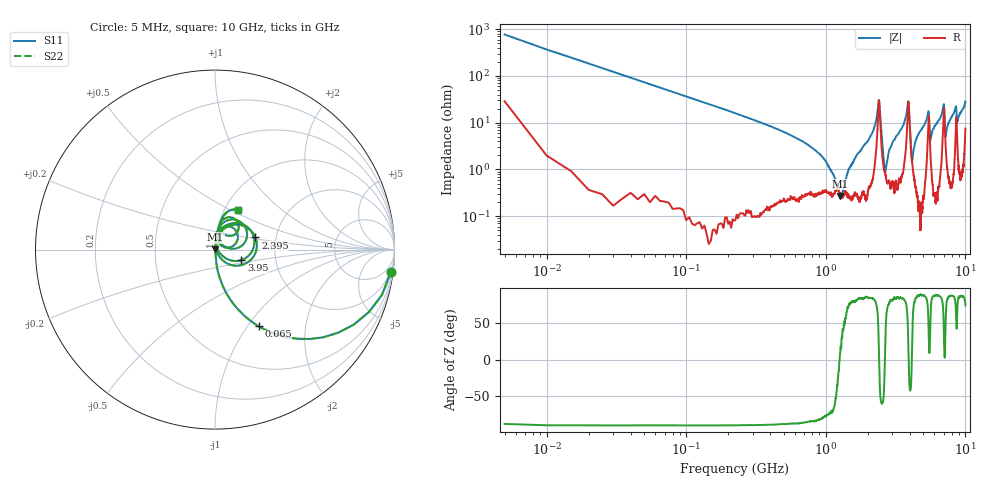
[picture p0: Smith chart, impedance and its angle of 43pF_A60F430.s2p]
! Amotech Co.,Ltd.
! http://www.amotech.co.kr/
! Part Number: A60F430
! These Parameters are Measured in Series Mode Connection
! Operation Temp=25[degC], DC Bias Voltage=0[V]
! Freq. Start=5[MHz] Stop=10[GHz], 2000[Steps]
! Date: Monday, July 20, 2020, 03:41:23
# GHZ S RI R 50.000000
!Freq.(Hz) S11(Real) S11(Imag) S21(Real) S21(Imag) S12(Real) S12(Imag) S22(Real) S22(Imag)
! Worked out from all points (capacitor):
!   2000 points, 5 MHz to 10 GHz, reference 50 ohm
!   read as one part in series: C = 43.3 pF near 55 MHz
!   lowest |Z| = 271 mohm at 1.27 GHz (marker M1)
!   series resonance near 1.256 GHz, so ESL is about 370 pH
!   S11 on the Smith chart (normalised r, x): 5 MHz: 2, -15; 65 MHz: 1.00, -1.13; 2.395 GHz: 1.56, +0.22; 3.95 GHz: 1.33, -0.16; 10 GHz: 1.15, +0.55
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0.005  0.9789 -0.1264  0.0211 0.1264  0.0211 0.1264  0.9789 -0.1264
0.065  0.2424 -0.4267  0.7576 0.4267  0.7576 0.4267  0.2424 -0.4267
0.22  0.0267 -0.1586  0.9733 0.1586  0.9733 0.1586  0.0267 -0.1586
0.955  0.00364 -0.0176  0.9964 0.0176  0.9964 0.0176  0.00364 -0.0176
1.27  0.00264 0.000585  0.9974 -0.000585  0.9974 -0.000585  0.00264 0.000585
1.675  0.00329 0.0204  0.9967 -0.0204  0.9967 -0.0204  0.00329 0.0204
2.395  0.2256 0.0676  0.7744 -0.0676  0.7744 -0.0676  0.2256 0.0676
2.66  0.00823 0.00204  0.9918 -0.00204  0.9918 -0.00204  0.00823 0.00204
2.875  0.00562 0.0271  0.9944 -0.0271  0.9944 -0.0271  0.00562 0.0271
3.34  0.01 0.0595  0.99 -0.0595  0.99 -0.0595  0.01 0.0595
3.87  0.1755 0.1293  0.8245 -0.1293  0.8245 -0.1293  0.1755 0.1293
3.95  0.1474 -0.0584  0.8526 0.0584  0.8526 0.0584  0.1474 -0.0584
4.155  0.0138 0.0057  0.9862 -0.0057  0.9862 -0.0057  0.0138 0.0057
5.005  0.00947 0.0829  0.9905 -0.0829  0.9905 -0.0829  0.00947 0.0829
5.43  0.1073 0.1156  0.8927 -0.1156  0.8927 -0.1156  0.1073 0.1156
5.615  0.0229 0.0333  0.9771 -0.0333  0.9771 -0.0333  0.0229 0.0333
6.67  0.0272 0.1297  0.9728 -0.1297  0.9728 -0.1297  0.0272 0.1297
7  0.1686 0.1247  0.8314 -0.1247  0.8314 -0.1247  0.1686 0.1247
7.21  0.0339 0.0343  0.9661 -0.0343  0.9661 -0.0343  0.0339 0.0343
8.335  0.041 0.1646  0.959 -0.1646  0.959 -0.1646  0.041 0.1646
8.75  0.0457 0.0876  0.9543 -0.0876  0.9543 -0.0876  0.0457 0.0876
10  0.1265 0.2228  0.8735 -0.2228  0.8735 -0.2228  0.1265 0.2228
